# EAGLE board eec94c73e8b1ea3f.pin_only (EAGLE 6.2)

Size 25.4 x 22.24 mm. Coordinates in mm from the lower left corner, seen from the top.
Outline: 0,2.54 0,19.7 arc-90 2.54,22.24 22.86,22.24 arc-90 25.4,19.7 25.4,2.54 arc-90 22.86,0 2.54,0 arc-90 0,2.54
Copper layers (1*16): Top 0.035mm / dielectric 1.5mm / Bottom 0.035mm
Design rules: minimum track width 8mil, minimum drill 0.4mm, track to track 8mil, track to pad 8mil, pad to pad 8mil, via to via 8mil, smd to smd 8mil, copper to edge 20mil, drill to drill 8mil, minimum pad ring 8mil, minimum via ring 10mil, stop-mask expansion 3mil, vias tented up to drill 0mil, thermal gap 8mil
bRestrict: area 10.2,2.5 to 10.3,3; area 8.3,2.5 to 8.4,3

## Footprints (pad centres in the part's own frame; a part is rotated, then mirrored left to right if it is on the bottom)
0805 = smd 1.3 x 1.5: 1 -0.95,0; 2 0.95,0
FIDUCIAL_1MM = smd 1 x 1: 1 0,0
1X2-3.5MM = drill 1 pad 2.184: 1 1.8,0; 2 -1.7,0
1X06_ROUND_70 = drill 1 pad 1.778: 1 -6.35,0; 2 -3.81,0; 3 -1.27,0; 4 1.27,0; 5 3.81,0; 6 6.35,0
2512 = smd 1.8 x 3.2: 1 -2.8,0; 2 2.8,0
SOLDERJUMPER_REFLOW_NOPASTE = smd 1.168 x 1.6: 1 -0.762,0; 2 0.762,0
SOT23-8 = smd 0.4 x 1.2: 1 -0.975,-1.3; 2 -0.325,-1.3; 3 0.325,-1.3; 4 0.975,-1.3; 5 0.975,1.3; 6 0.325,1.3; 7 -0.325,1.3; 8 -0.975,1.3
MOUNTINGHOLE_2.5_PLATED = drill 2.5 pad 3.2: P$1 0,0

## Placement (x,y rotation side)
C1  0.1µF  [0805]  4.01,8.38 270 top
FID1  FIDUCIAL""  [FIDUCIAL_1MM]  23.01,16.46 0 top
FID2  FIDUCIAL""  [FIDUCIAL_1MM]  1.14,5.59 0 top
J1  TERMBLOCK_1X2-3.5MM  [1X2-3.5MM]  12.8,18.9 180 top
JP1  [1X06_ROUND_70]  13.08,2.79 0 top
R1  10K  [0805]  18.29,6.86 0 top
R2  10K  [0805]  18.29,9.39 0 top
R3  10K  [0805]  6.55,8.38 90 top
R4  10K  [0805]  8.89,8.38 90 top
R5  0.1/1% (PT2512FK-070R1L)  [2512]  12.7,13.54 0 top
SJ1  [SOLDERJUMPER_REFLOW_NOPASTE]  22.1,6.86 180 top
SJ2  [SOLDERJUMPER_REFLOW_NOPASTE]  22.1,9.39 180 top
U1  INA219BIDCNT  [SOT23-8]  12.7,8.38 180 top
U$7  MOUNTINGHOLE2.5  [MOUNTINGHOLE_2.5_PLATED]  22.86,2.54 0 top
U$8  MOUNTINGHOLE2.5  [MOUNTINGHOLE_2.5_PLATED]  2.54,2.54 0 top
U$9  MOUNTINGHOLE2.5  [MOUNTINGHOLE_2.5_PLATED]  2.54,19.7 0 top
U$10  MOUNTINGHOLE2.5  [MOUNTINGHOLE_2.5_PLATED]  22.86,19.7 0 top
U$11  [ADAFRUIT_3.5MM]  17.17,14.18 0 top

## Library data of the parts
C1 FID1 FID2 J1 JP1 R1-R5 SJ1 SJ2 U1 U$7-U$11 = microbuilder

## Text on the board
tPlace: Vin- | Vin+ | INA219 DC | Current | Sensor | R5 | I2C Address | A1 | A0 | Gnd | Sda | Vin+ | Vcc | Scl | Vin-
bPlace: INA219 DC Current | Monitor | Bus Voltage: 0-26V | Max Current: 3.2A | VCC/LOGIC: 3-5V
